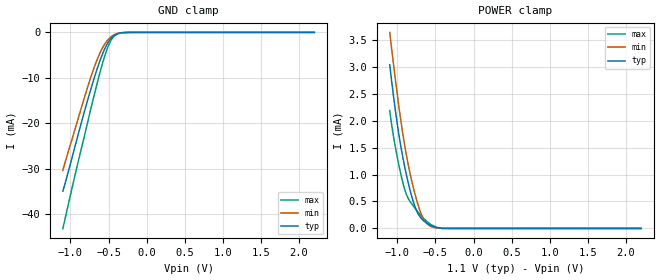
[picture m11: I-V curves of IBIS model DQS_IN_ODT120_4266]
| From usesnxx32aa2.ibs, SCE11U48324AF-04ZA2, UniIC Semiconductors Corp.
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| DQS_IN_ODT120_4266 (with 120ohm ODT, 3200-4266Mbps)
[Model]   DQS_IN_ODT120_4266
Model_type   Input
Vinl = 123.333mV
Vinh = 243.333mV
|   typ   min   max
|C_comp   0.825pF   0.777pF   0.876pF
C_comp_power_clamp   0.4125pF   0.3885pF   0.4380pF
C_comp_gnd_clamp   0.4125pF   0.3885pF   0.4380pF
| Note: C_comp changes when the ODT circuit is enabled.
[Model Spec]
| Input threshold voltage corners
Vinl   0.1233V   0.1167V   0.1350V
Vinh   0.2433V   0.2367V   0.2550V
| Dynamic Overshoot Parameters from LPDDR4 Specification
D_overshoot_ampl_h   0.30   NA   NA
D_overshoot_ampl_l   0.30   NA   NA
D_overshoot_area_h   0.1n   NA   NA
D_overshoot_area_l   0.1n   NA   NA
[Receiver Thresholds]
Vcross_low   = 123.3mV
Vcross_high  = 243.3mV
Vdiff_ac   = 120mV
Vdiff_dc   = 120mV
Tdiffslew_ac = 10.000ns |Not specified, so set to high value
[Voltage Range]   1.1000V   1.0600V   1.1700V
[POWER Clamp Reference]   1.1000V   1.0600V   1.1700V
| Junction Temperature (Ambient temp is 35C typ 95C min -40C max)
[Temperature Range]   50.0   110.0   -40.0
[Add Submodel]
| Submodel Name   Mode
120ohm_ODT_4266   Non-Driving
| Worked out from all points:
|   GND clamp passes 1 mA (typ) near -0.45 V on its own axis
|   POWER clamp passes 1 mA (typ) near -0.88 V on its own axis
[GND Clamp]
|   Voltage   I(typ)   I(min)   I(max)
-1.1V     -34.88mA   -30.34mA   -43.13mA
-941.6mV  -25.13mA   -21.34mA   -31.47mA
-789.8mV  -15.79mA   -12.83mA   -20.82mA
-727.1mV  -12.17mA   -9.549mA   -16.41mA
-661.1mV  -8.598mA   -6.455mA   -11.9mA
-591.8mV  -5.273mA   -3.798mA   -7.529mA
-522.5mV  -2.672mA   -1.912mA   -3.822mA
-463.1mV  -1.24mA    -904.9uA   -1.604mA
-407mV    -507uA     -377.3uA   -542.1uA
-334.4mV  -115.1uA   -86.84uA   -97.76uA
-218.9mV  -5.347uA   -5.058uA   -2.413uA
2.2V      0A         0A         0A
[POWER Clamp]
|   Voltage   I(typ)   I(min)   I(max)
-1.1V     3.036mA    3.636mA    2.186mA
-1.041V   2.347mA    2.931mA    1.626mA
-977.9mV  1.724mA    2.242mA    1.161mA
-905.3mV  1.155mA    1.554mA    733uA
-849.2mV  799.6uA    1.127mA    536.8uA
-776.6mV  434.3uA    683.8uA    390.2uA
-710.6mV  233.6uA    359.2uA    273.1uA
-651.2mV  137.4uA    162.5uA    181.2uA
-591.8mV  78.18uA    65.06uA    105.7uA
-496.1mV  17.57uA    12.35uA    25.98uA
-377.3mV  3.689uA    1.066uA    1.269uA
2.2V      0A         0A         0A
